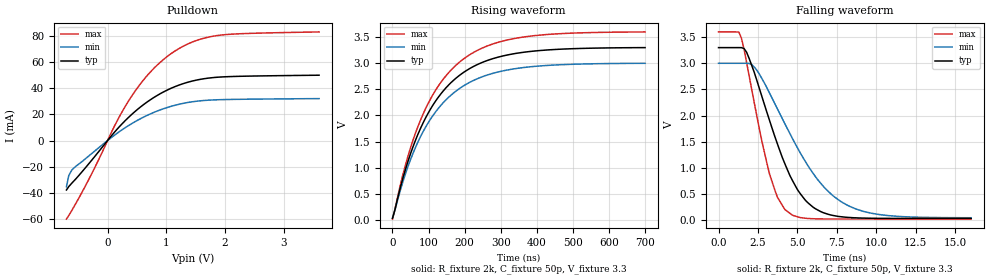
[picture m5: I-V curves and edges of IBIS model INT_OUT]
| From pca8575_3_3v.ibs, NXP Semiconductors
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[Model]   INT_OUT
Model_type Open_drain
Vref=3.3
Vmeas=1.65
Rref=2k
Cref=50p
C_comp   5.4p   5.2p   5.7p
[Temperature Range] 27   85   -40
[Voltage Range]   3.3   3   3.6
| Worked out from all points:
|   slope of the pulldown table from 0 to 0.495 V, typ, clamps not added: 21.3 ohm
|   falling waveform, R_fixture 2k, C_fixture 50p, V_fixture 3.3: 20-80 % time 2.36ns typ, 3.4ns min, 1.53ns max; typ from 3.3 V to 0.029 V
|   rising waveform, R_fixture 2k, C_fixture 50p, V_fixture 3.3: 20-80 % time 140ns typ, 141ns min, 140ns max; typ from 0.029 V to 3.3 V
[Pulldown]
-700mV    -37.76mA   -35.32mA   -59.97mA
-660mV    -35.15mA   -26.69mA   -57.21mA
-570mV    -30.74mA   -20.83mA   -50.41mA
-270mV    -15.02mA   -9.931mA   -25.35mA
130mV     7.014mA    4.501mA    12.16mA
340mV     16.96mA    10.97mA    29.02mA
520mV     24.18mA    15.72mA    40.98mA
690mV     29.97mA    19.56mA    50.43mA
1.04V     39.08mA    25.58mA    65.04mA
1.43V     45.31mA    29.53mA    75.03mA
1.82V     48.17mA    31.07mA    79.89mA
3.6V      49.91mA    32.03mA    82.97mA
[Falling Waveform]
R_fixture=2k
C_fixture=50p
V_fixture=3.3
V_fixture_min=3
V_fixture_max=3.6
0s        3.3V       3V         3.6V
1.455ns   3.299V     3V         3.477V
2.263ns   2.828V     2.928V     2.248V
3.232ns   1.906V     2.43V      880mV
3.717ns   1.469V     2.135V     444mV
4.687ns   753.7mV    1.557V     91.37mV
6.141ns   214.6mV    829mV      22.34mV
8.242ns   48.77mV    269.8mV    18.35mV
10.67ns   30.62mV    86.64mV    18.3mV
16ns      29.3mV     42.72mV    18.3mV
[Rising Waveform]
R_fixture=2k
C_fixture=50p
V_fixture=3.3
V_fixture_min=3
V_fixture_max=3.6
0s        29.3mV     41.6mV     18.3mV
21.21ns   603mV      553.2mV    653.5mV
42.42ns   1.11V      1.012V     1.209V
63.64ns   1.523V     1.386V     1.66V
84.85ns   1.858V     1.69V      2.026V
134.3ns   2.414V     2.195V     2.634V
198ns     2.827V     2.57V      3.085V
268.7ns   3.064V     2.785V     3.344V
360.6ns   3.205V     2.913V     3.497V
700ns     3.297V     2.997V     3.596V
[Ramp]
R_load=2k
dV/dt_r   1.962E+0/2.292E-9   1.952E+0/2.527E-9   1.970E+0/2.035E-9
dV/dt_f   1.962E+0/1.351E-10   1.953E+0/2.447E-10   1.970E+0/7.871E-11
|[End   INT_OUT
